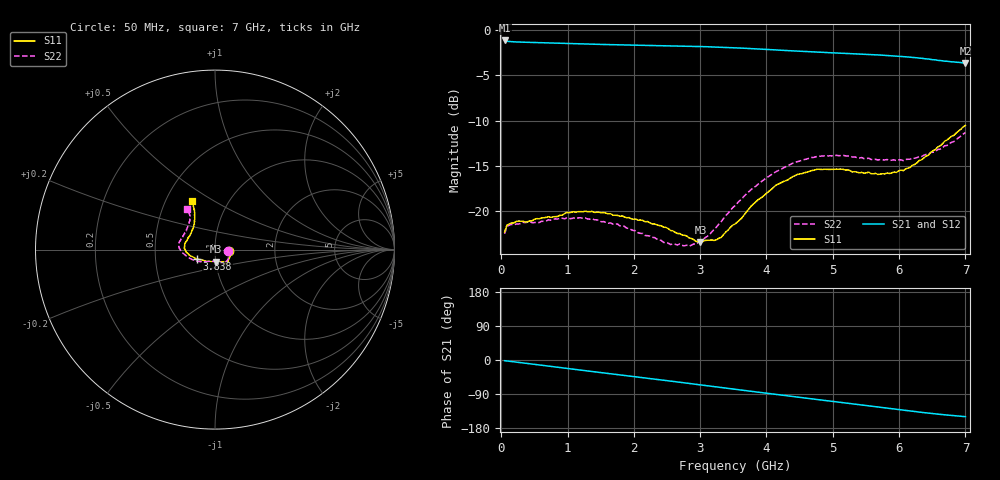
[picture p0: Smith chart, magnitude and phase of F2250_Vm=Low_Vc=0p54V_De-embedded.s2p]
! Integrated Device Technology
! Corporate Headquarters
! 6024 Silver Creek Valley Road
! San Jose, CA 95138  USA
! Phone:  1-408-284-8200
! Toll Free:  1-800-223-1366
! Webpage:  http://www.idt.com/
! Timing and RF Division
! 515 Groton Road, Suite 102
! Westford, MA 01886-6024
! Device:  F2250
! Description: Voltage Variable RF Attenuator
! Frequency:  50.0 -  6000.00 MHz
! Package:  3x3 mm Thin QFN Plastic Package: 16 pin
! Ports:  2 RF, 3 DC
!  Pin  1  = GND
!  Pin  2  = NC
!  Pin  3  = RF1  = Port 1
!  Pin  4  = NC
!  Pin  5  = GND
!  Pin  6  = GND
!  Pin  7  = GND
!  Pin  8  = GND
!  Pin  9  = NC
!  Pin 10  = RF2  = Port 2
!  Pin 11  = NC
!  Pin 12  = GND
!  Pin 13  = GND
!  Pin 14  = VCNTRL
!  Pin 15  = VDD
!  Pin 16  = VMODE
! Vcntrl:  0.540 Volts
! Vmode:  +0.000 Volts
! Vdd:  +3.30  Volts
! Current:  1.133 mA
! Data:  The device was measured on a the F2250 evaluation board which has
!  individual transmission lines to the RF pins.  Data was collected
!  using a calibrated network analyzer.  The evaluation board was
!  de-embedded using a TRL calibration technique.
!  The reference plane is the edge of the package pin.
! Misc:  SN 10
!  Action Tracker AT0258
! Date Measured:  2014-11-26
! Date:  2015-10-15  MJV
! Note:
!  Integrated Device Technology supplies this data as a sample of measured
!  data at the package pin for this product.  Your particular data for this
!  product may vary.
!  Data was taken at 25 degrees C.
!  Integrated Device Technology reserves the right to change this data at anytime.
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# GHz S dB R 50
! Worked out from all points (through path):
!   201 points, 50 MHz to 7 GHz, reference 50 ohm
!   highest |S21| = -1.13 dB at 50 MHz (marker M1); lowest = -3.6 dB at 7 GHz (marker M2)
!   group delay of S21, straight-line fit = 60.1 ps
!   lowest |S11| = -23.4 dB at 3.004 GHz (marker M3), VSWR 1.15, Z = 50.1 - j6.81 ohm
!   |S11| at or under -10 dB: start of sweep to end of sweep
!   |S22| runs from -23.8 to -11.3 dB; largest |S21 - S12| = 0.0004
!   S11 on the Smith chart (normalised r, x): 50 MHz: 1.16, -0.02; 3.838 GHz: 0.81, -0.09; 7 GHz: 0.68, +0.40
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0.05  -22.28 -7.2  -1.13 -1.8  -1.13 -1.8  -22.48 -8.1
0.08475  -21.52 -7.2  -1.22 -2.5  -1.22 -2.5  -21.67 -7.6
0.15425  -21.28 -9.3  -1.27 -4.0  -1.27 -4.0  -21.44 -9.4
0.71025  -20.59 -31.5  -1.41 -16.2  -1.40 -16.2  -20.93 -34.5
1.2315  -20.04 -47.7  -1.52 -27.4  -1.52 -27.4  -20.77 -54.6
1.75275  -20.44 -54.5  -1.61 -38.5  -1.61 -38.5  -21.38 -63.7
2.37825  -21.55 -56.6  -1.70 -51.8  -1.70 -51.8  -23.14 -70.7
2.552  -22.10 -60.1  -1.72 -55.6  -1.72 -55.6  -23.66 -76.6
2.83  -22.91 -71.6  -1.77 -61.7  -1.77 -61.7  -23.83 -92.9
3.00375  -23.36 -85.2  -1.81 -65.6  -1.80 -65.6  -23.23 -106.2
3.14275  -23.17 -96.5  -1.84 -68.6  -1.84 -68.6  -22.55 -117.8
3.3165  -22.87 -115.1  -1.88 -72.5  -1.88 -72.5  -21.13 -129.6
3.525  -21.39 -132.9  -1.95 -77.2  -1.94 -77.2  -19.37 -141.7
3.83775  -18.95 -152.1  -2.06 -84.1  -2.06 -84.1  -17.22 -156.0
4.1505  -17.07 -165.2  -2.19 -90.9  -2.19 -91.0  -15.59 -168.3
4.7065  -15.47 179.1  -2.40 -103.0  -2.40 -103.0  -14.05 177.7
5.15825  -15.37 168.1  -2.56 -112.7  -2.56 -112.7  -13.81 168.2
5.85325  -15.82 144.3  -2.80 -127.6  -2.80 -127.7  -14.38 152.5
6.166  -15.15 132.5  -2.97 -134.4  -2.97 -134.5  -14.24 143.5
6.444  -13.79 123.2  -3.18 -140.2  -3.18 -140.3  -13.69 134.0
6.82625  -11.60 116.6  -3.50 -146.9  -3.50 -146.9  -12.29 125.9
7  -10.51 115.7  -3.62 -149.6  -3.62 -149.6  -11.31 124.3
